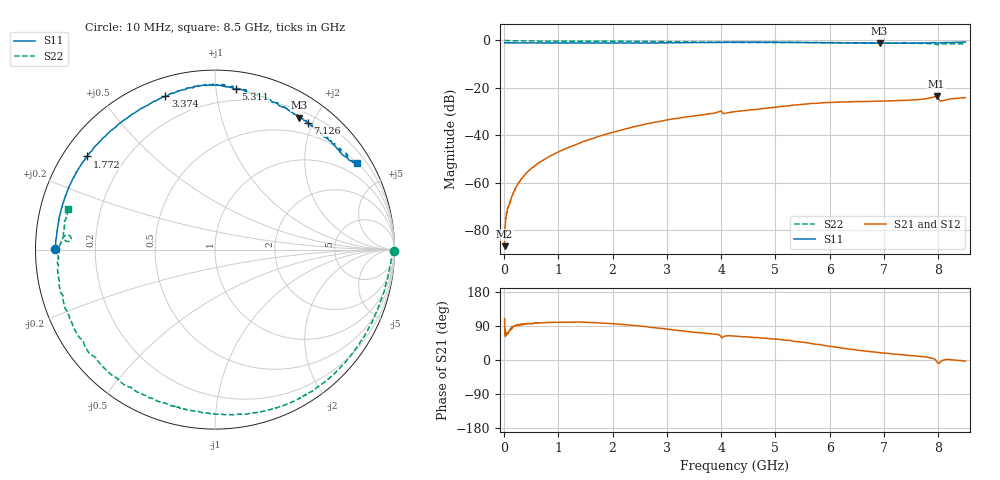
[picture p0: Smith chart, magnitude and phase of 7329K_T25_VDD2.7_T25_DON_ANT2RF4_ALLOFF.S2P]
!Agilent Technologies,E5071C,MY46417908,A.11.23
!Date: Mon Aug 31 18:03:36 2020
!Data & Calibration Information:
!Freq	S11:SOLT2(ON)	S21:SOLT2(ON)	S12:SOLT2(ON)	S22:SOLT2(ON)
!PortZ  Port1:50+j0  Port2:50+j0
!Above PortZ is port z conversion or system Z0 setting when saving the data.
!When reading, reference impedance value at option line is always used.
# Hz S dB R 50
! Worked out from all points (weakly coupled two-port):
!   1601 points, 10 MHz to 8.5 GHz, reference 50 ohm
!   highest |S21| = -23.54 dB at 7.969 GHz (marker M1); lowest = -86.6 dB at 10 MHz (marker M2)
!   lowest |S11| = -1.2 dB at 6.919 GHz (marker M3), VSWR 14.67, Z = 14.5 + j89.4 ohm
!   |S11| at or under -10 dB: nowhere
!   |S22| runs from -1.9 to 0.0 dB; largest |S21 - S12| = 0.001
!   S11 on the Smith chart (normalised r, x): 10 MHz: 0.06, +0.00; 1.772 GHz: 0.07, +0.32; 3.374 GHz: 0.08, +0.72; 5.311 GHz: 0.11, +1.13; 7.126 GHz: 0.32, +1.93; 8.5 GHz: 0.50, +3.48
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1e7  -0.99 179.7  -86.65 109.2  -85.62 70.5  -0.02 -0.4
7.3675e7  -1.02 178.1  -70.38 70.1  -71.09 73.2  -0.11 -2.2
1.58575e8  -1.03 176.1  -65.10 85.9  -64.59 85.5  -0.15 -4.1
2.753125e8  -1.06 173.3  -59.88 94.0  -59.61 93.7  -0.20 -6.6
4.13275e8  -1.06 170.2  -55.79 96.0  -55.90 96.4  -0.22 -9.9
8.271625e8  -1.06 161.5  -48.95 99.1  -49.02 99.2  -0.30 -19.1
1.426769e9  -1.06 150.7  -42.94 100.1  -42.93 100.2  -0.36 -33.3
1.771675e9  -1.09 144.0  -40.21 97.8  -40.22 97.7  -0.37 -41.5
2.843538e9  -1.06 119.4  -34.19 84.1  -34.19 84.1  -0.46 -67.1
3.374162e9  -0.94 107.9  -32.16 75.4  -32.15 75.5  -0.63 -80.6
3.968462e9  -0.79 98.2  -29.91 65.8  -29.90 65.8  -0.84 -95.6
4.069281e9  -0.77 97.5  -30.74 63.1  -30.74 63.1  -0.85 -97.5
4.255e9  -0.76 95.4  -30.00 63.2  -29.99 63.1  -0.87 -101.9
5.310944e9  -0.87 82.6  -27.31 50.5  -27.28 50.6  -0.90 -126.6
5.671769e9  -0.95 76.8  -26.55 43.1  -26.51 43.3  -0.94 -137.6
6.345662e9  -1.04 66.8  -25.88 29.4  -25.95 29.7  -0.96 -159.8
6.918738e9  -1.19 57.5  -25.60 19.4  -25.65 19.2  -1.07 -172.7
7.088538e9  -1.14 54.6  -25.50 17.3  -25.56 17.0  -1.10 -175.0
7.125681e9  -1.16 53.8  -25.47 16.6  -25.50 16.5  -1.10 -175.5
7.969375e9  -1.03 38.6  -23.54 -3.1  -23.56 -2.8  -1.69 174.4
8.070194e9  -0.98 35.4  -25.45 -1.5  -25.47 -1.6  -1.53 176.3
8.5e9  -0.66 31.5  -24.05 -2.8  -24.14 -3.1  -1.42 164.6
